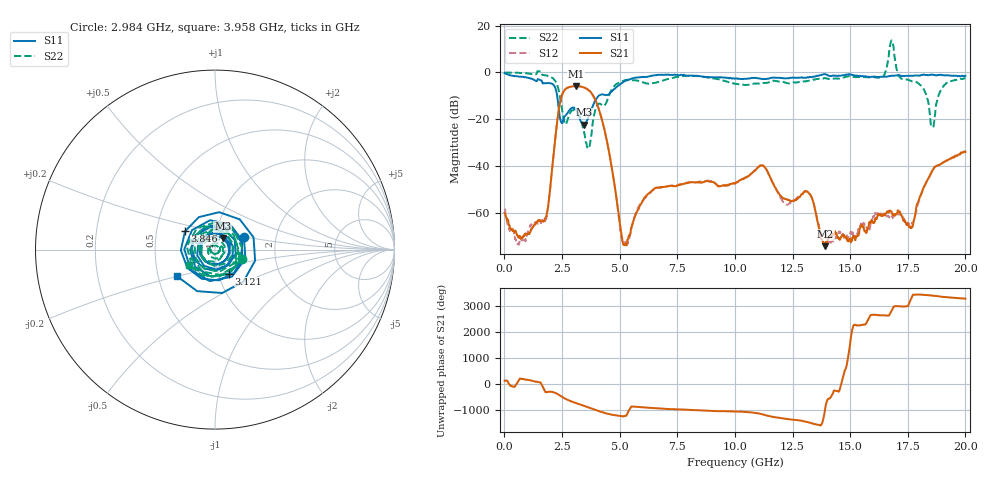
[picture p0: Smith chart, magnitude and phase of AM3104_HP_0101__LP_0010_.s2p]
!Created with skrf (http://scikit-rf.org).
# Hz S RI R 50.0
!freq ReS11 ImS11 ReS21 ImS21 ReS12 ImS12 ReS22 ImS22
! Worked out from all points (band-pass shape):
!   1601 points, 10 MHz to 20 GHz, reference 50 ohm
!   highest |S21| = -5.81 dB at 3.108 GHz (marker M1); lowest = -74.2 dB at 13.93 GHz (marker M2)
!   |S21| within 3 dB of the highest: 2.531 GHz to 3.776 GHz (1.245 GHz wide, 39.5 % of centre)
!   lowest |S11| = -22.3 dB at 3.458 GHz (marker M3), VSWR 1.17, Z = 54 + j6.87 ohm
!   |S11| at or under -10 dB: 2.29 GHz to 4.081 GHz (1.791 GHz wide, 56.2 % of centre)
!   |S22| runs from -32.5 to 13.7 dB; largest |S21 - S12| = 0.029
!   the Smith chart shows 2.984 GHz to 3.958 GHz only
!   S11 on the Smith chart (normalised r, x): 2.984 GHz: 1.37, +0.20; 3.121 GHz: 1.13, -0.31; 3.846 GHz: 0.70, +0.15; 3.958 GHz: 0.63, -0.20
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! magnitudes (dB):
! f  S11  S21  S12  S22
! 10 MHz  -0.3  -59.9  -58.1  -0.1
! 559.7 MHz  -1.6  -69.4  -72.7  -0.1
! 1.772 GHz  -4.6  -62.3  -63.3  -1.2
! 2.421 GHz  -19.8  -12.5  -12.5  -10.7
! 2.984 GHz  -15.1  -5.9  -5.9  -16.1
! 3.108 GHz  -16.1  -5.8  -5.8  -16.8
! 3.121 GHz  -16.2  -5.8  -5.8  -17.1
! 3.346 GHz  -21.4  -6.1  -6.1  -20.8
! 3.458 GHz  -22.3  -6.4  -6.4  -25.5
! 3.846 GHz  -14.2  -9.8  -9.8  -20.6
! 3.958 GHz  -11.7  -12.0  -12.0  -15.5
! 5.207 GHz  -3.7  -73.4  -72.8  -3.4
! 6.682 GHz  -1.0  -49.2  -49.1  -4.1
! 10.01 GHz  -2.7  -47.4  -47.4  -4.8
! 11.18 GHz  -2.8  -39.7  -39.8  -4.6
! 12.19 GHz  -2.5  -54.0  -56.3  -4.3
! 13.34 GHz  -2.0  -53.4  -53.7  -3.3
! 13.93 GHz  -0.7  -74.2  -69.4  -2.4
! 16.68 GHz  -1.6  -59.8  -61.6  7.2
! 17.64 GHz  -1.4  -66.0  -65.0  -3.6
! 18.56 GHz  -0.9  -41.9  -42.1  -23.3
! 20 GHz  -1.4  -33.9  -33.6  -2.5
